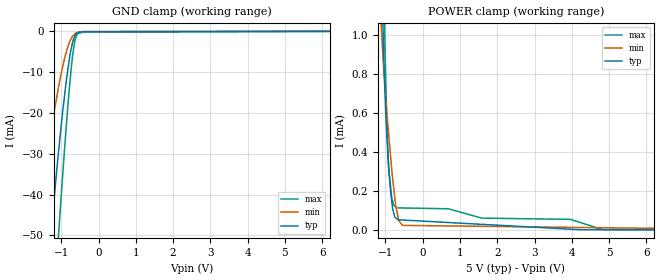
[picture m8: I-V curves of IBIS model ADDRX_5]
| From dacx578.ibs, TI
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|   ADDRX Model 5V MODEL
[Model] ADDRX_5
Model_type   Input
Vinl = 1.5
Vinh = 3.5
|   typ   min   max
|   (Nom PVT)   (Fast PVT)  (Slow PVT)
C_comp   3.0371940e-12   2.5153120e-12   3.5888940e-12
|Where nom PVT is Nom process, 5.0V, 27C
|Fast PVT is Strong Process, 5.5V, -40C
|Slow PVT is Weak Process,   4.5V, 125C
[Voltage Range]   5   4.5   5.5
[Temperature Range]   27   125   -40
|Junction temperatures are used for [Temperature Range]
[Power Clamp Reference]   5   4.5   5.5
[GND Clamp Reference]   0   0   0
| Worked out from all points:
|   GND clamp passes 1 mA (typ) near -0.62 V on its own axis
|   POWER clamp passes 1 mA (typ) near -1.06 V on its own axis
[GND Clamp]
|   Voltage   I(typ)   I(min)   I(max)
-5V       -510.8mA   -352.1mA   -618.9mA
-1.677V   -94.23mA   -50.71mA   -135.4mA
-1.575V   -82.39mA   -43.43mA   -120.6mA
-1.265V   -48.43mA   -23.9mA    -76.23mA
-1.083V   -30.42mA   -14.22mA   -51.2mA
-1.059V   -28.23mA   -12.95mA   -47.86mA
-871.1mV  -12.56mA   -5.317mA   -23.9mA
-727.8mV  -4.057mA   -1.75mA    -8.632mA
-685.1mV  -2.428mA   -1.166mA   -5.235mA
-627.7mV  -1.09mA    -631.9uA   -2.139mA
-524.2mV  -251.6uA   -232.6uA   -536.4uA
9.985V    0A         0A         0A
[POWER Clamp]
|   Voltage   I(typ)   I(min)   I(max)
-5V       47.04mA    36.93mA    57.5mA
-1.118V   1.439mA    1.065mA    2.084mA
-1.066V   1.035mA    884.9uA    1.488mA
-1.036V   825.5uA    796.8uA    1.178mA
-1.014V   709.5uA    737.7uA    954.3uA
-966.9mV  500.1uA    610.4uA    575.8uA
-926.9mV  357uA      517.8uA    367.5uA
-830.7mV  147.1uA    308.7uA    165.9uA
-719.3mV  61.11uA    118.2uA    116.3uA
-542.1mV  51.07uA    23.45uA    112.8uA
4.81V     1.288uA    11.53uA    3.033uA
9.985V    0A         0A         0A
